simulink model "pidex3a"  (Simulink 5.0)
settings: Solver=ode45  StartTime=0.0  StopTime=2

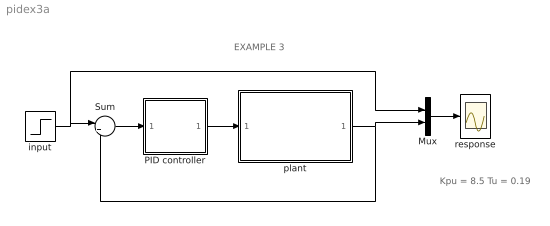
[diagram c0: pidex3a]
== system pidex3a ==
  note: EXAMPLE 3
  note: Kpu = 8.5 Tu = 0.19
  Mux : Mux  Inputs=2
  PID controller : Subsystem  mask{Kp=5.1, Ki=53.7, Kd=0.11, sat=2}
      mask prompts: Kp "Proportional gain (Kp)"; Ki "Integral gain (Ki)"; Kd "Derivative gain (Kd)"; sat "Saturation limit [pu]"
      mask help: Proportional-Integral Speed Controller
  Sum : Sum  Inputs=|+-
  input : Step  Time=.05  SampleTime=0
  plant : Subsystem  mask{Ka=1, Ta=0.25, Td=0.05}
      mask prompts: Ka "Gain"; Ta "Time constant [s]"; Td "Time delay [s]"
  response : Scope
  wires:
  plant/1(Out1) -> Sum/2, Mux/2
  Sum/1 -> PID controller/1(er)
  PID controller/1(c) -> plant/1(In1)
  input/1 -> Sum/1, Mux/1
  Mux/1 -> response/1

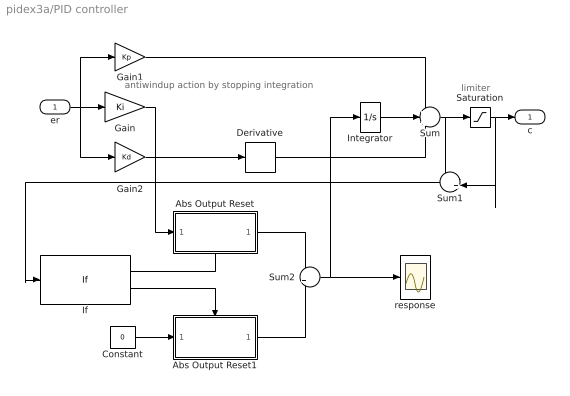
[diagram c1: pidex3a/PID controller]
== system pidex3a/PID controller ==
  note: antiwindup action by stopping integration
  note: limiter
  er : Inport
  Abs Output Reset : Subsystem  TreatAsAtomicUnit=on
  Abs Output Reset1 : Subsystem  TreatAsAtomicUnit=on
  Constant : Constant  Value=0
  Derivative : Derivative
  Gain : Gain  Gain=Ki
  Gain1 : Gain  Gain=Kp
  Gain2 : Gain  Gain=Kd
  If : If  IfExpression=u1<0
  Integrator : Integrator
  Saturation : Saturate  UpperLimit=sat  LowerLimit=-sat
  Sum : Sum  Inputs=+++
  Sum1 : Sum  Orientation=left  Inputs=-+
  Sum2 : Sum
  response : Scope
  c : Outport  InitialOutput=0
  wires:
  Gain1/1 -> Sum/1
  er/1 -> Gain1/1, Gain2/1, Gain/1
  Derivative/1 -> Sum/3
  Gain2/1 -> Derivative/1
  Sum/1 -> Saturation/1, Sum1/1
  Saturation/1 -> c/1, Sum1/2
  Integrator/1 -> Sum/2
  If/2 -> Abs Output Reset1/Action
  Constant/1 -> Abs Output Reset1/1(In)
  If/1 -> Abs Output Reset/Action
  Abs Output Reset/1(Out) -> Sum2/1
  Abs Output Reset1/1(Out) -> Sum2/2
  Gain/1 -> Abs Output Reset/1(In)
  Sum2/1 -> Integrator/1, response/1
  Sum1/1 -> If/1

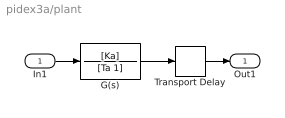
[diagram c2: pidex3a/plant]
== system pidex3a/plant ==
  In1 : Inport
  G(s) : TransferFcn  Numerator=[Ka]  Denominator=[Ta 1]
  Transport Delay : TransportDelay  DelayTime=Td  BufferSize=2048
  Out1 : Outport
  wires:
  G(s)/1 -> Transport Delay/1
  In1/1 -> G(s)/1
  Transport Delay/1 -> Out1/1

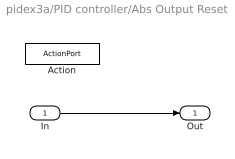
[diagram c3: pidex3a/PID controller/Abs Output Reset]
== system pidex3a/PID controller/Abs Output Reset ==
  In : Inport
  Action : ActionPort  InitializeStates=reset  ActionType=then
  Out : Outport  OutputWhenDisabled=reset  InitialOutput=0
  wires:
  In/1 -> Out/1

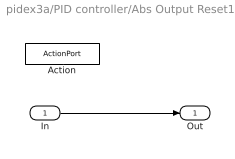
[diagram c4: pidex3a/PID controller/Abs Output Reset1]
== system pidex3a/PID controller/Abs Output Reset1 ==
  In : Inport
  Action : ActionPort  InitializeStates=reset  ActionType=else
  Out : Outport  OutputWhenDisabled=reset  InitialOutput=0
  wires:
  In/1 -> Out/1
